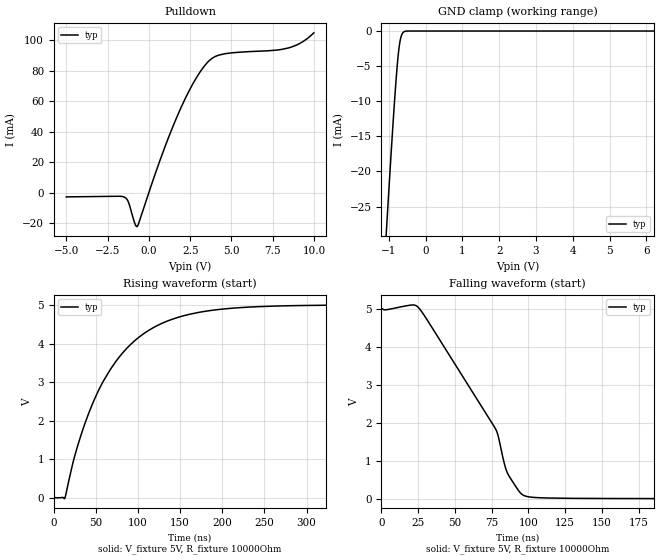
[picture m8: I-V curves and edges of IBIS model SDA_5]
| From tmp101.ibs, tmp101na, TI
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|   SDA 5 V Model
[Model]   SDA_5
Model_type   I/O_open_drain
Polarity   Non-Inverting
Enable   Active-Low
Vinl = 1.5
Vinh = 3.5
Vmeas = 2.5
Vref = 2.5
Cref = 15pF
Rref = 10000
|   typ   min   max
C_comp   4.925pF   NA   NA
[Voltage Range]   5   NA   NA
[Temperature Range]   27   NA   NA
[Pullup Reference]   5   NA   NA
[Pulldown Reference]   0   NA   NA
[Power Clamp Reference]   5   NA   NA
[GND Clamp Reference]   0   NA   NA
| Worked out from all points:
|   slope of the pulldown table from 0 to 0.75 V, typ, clamps not added: 32.1 ohm
|   GND clamp passes 1 mA (typ) near -0.67 V on its own axis
|   falling waveform, V_fixture 5V, R_fixture 10000Ohm: 20-80 % time 40.6ns typ, NA min, NA max; typ from 5 V to 0.015 V
|   rising waveform, V_fixture 5V, R_fixture 10000Ohm: 20-80 % time 68.6ns typ, NA min, NA max; typ from 0.015 V to 5 V
[Pulldown]
|   Voltage   I(typ)   I(min)   I(max)
-5V       -2.772mA   NA         NA
-1.492V   -2.883mA   NA         NA
-1.252V   -5.765mA   NA         NA
-854mV    -19.93mA   NA         NA
-711mV    -22.23mA   NA         NA
667.5mV   20.96mA    NA         NA
1.69V     49.41mA    NA         NA
2.662V    71.29mA    NA         NA
3.537V    85.23mA    NA         NA
4.585V    90.99mA    NA         NA
8.427V    94.77mA    NA         NA
9.985V    104.7mA    NA         NA
[GND Clamp]
|   Voltage   I(typ)   I(min)   I(max)
-5V       -388mA     NA         NA
-1.061V   -28.39mA   NA         NA
-1.038V   -26.31mA   NA         NA
-957.8mV  -19.43mA   NA         NA
-871.4mV  -12.31mA   NA         NA
-810.8mV  -7.745mA   NA         NA
-758.6mV  -4.351mA   NA         NA
-718.5mV  -2.365mA   NA         NA
-674.3mV  -1.016mA   NA         NA
-628.6mV  -361.2uA   NA         NA
-568.7mV  -65.99uA   NA         NA
9.985V    0A         NA         NA
[POWER Clamp]
|   SCR cell for ESD function. Effects occurr above VDD x 2
|   Voltage   I(typ)   I(min)   I(max)
-5V       0A         0A         0A
0V        0A         0A         0A
10V       0A         0A         0A
[Ramp]
R_load = 10000
|   typ   min   max
dV/dt_r   2.99082/6.85943e-008 NA   NA
dV/dt_f   2.99082/4.05535e-008 NA   NA
[Falling Waveform]
V_fixture = 5V
R_fixture = 10000Ohm
C_fixture = 0F
|   Time   V(typ)   V(min)   V(max)
0s        5V         NA         NA
21.62ns   5.099V     NA         NA
25.94ns   5.001V     NA         NA
77.79ns   1.841V     NA         NA
79.56ns   1.652V     NA         NA
84.13ns   875.5mV    NA         NA
86.92ns   608.9mV    NA         NA
94.92ns   155.5mV    NA         NA
102.1ns   55.05mV    NA         NA
1.201us   15.28mV    NA         NA
[Rising Waveform]
V_fixture = 5V
R_fixture = 10000Ohm
C_fixture = 0F
|   Time   V(typ)   V(min)   V(max)
0s        15.3mV     NA         NA
13.06ns   -4.422mV   NA         NA
24.58ns   1.069V     NA         NA
41.37ns   2.192V     NA         NA
57.93ns   2.992V     NA         NA
77.47ns   3.645V     NA         NA
116.6ns   4.392V     NA         NA
173ns     4.81V      NA         NA
320.9ns   4.991V     NA         NA
1.201us   5V         NA         NA
